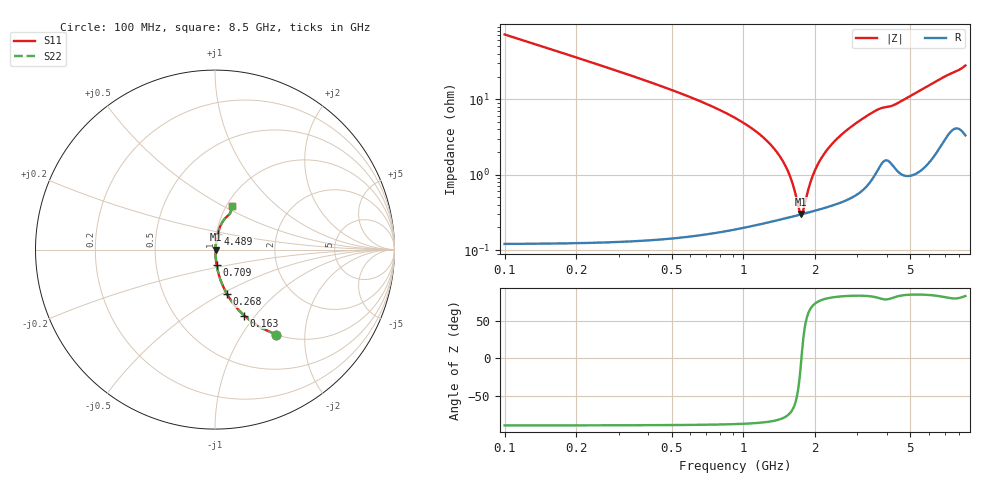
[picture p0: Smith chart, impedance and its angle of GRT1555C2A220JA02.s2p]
!Murata Part Number: GRT1555C2A220JA02
!These Parameters are Measured in Series Mode Connection
!Data Generated on Jun 19, 2026
!  o--ll--o
!Port1  Port2
!  o------o
!Operation Temp=25[degC], DC Bias Voltage=0[V]
!Freq. Start=100[MHz] Stop=9[GHz] 401[Steps]
# Hz S RI R 50
!Freq.(Hz) S11(Real) S11(Imag) S21(Real) S21(Imag) S12(Real) S12(Imag) S22(Real) S22(Imag)
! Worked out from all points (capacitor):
!   401 points, 100 MHz to 8.5 GHz, reference 50 ohm
!   read as one part in series: C = 22 pF near 142 MHz
!   lowest |Z| = 302 mohm at 1.738 GHz (marker M1)
!   series resonance near 1.749 GHz, so ESL is about 380 pH
!   S11 on the Smith chart (normalised r, x): 100 MHz: 1.00, -1.44; 163 MHz: 1.00, -0.88; 268 MHz: 1.00, -0.53; 709 MHz: 1.00, -0.17; 4.489 GHz: 1.02, +0.18; 8.5 GHz: 1.07, +0.56
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1e8  0.3423 -0.4736  0.6577 0.4736  0.6577 0.4736  0.3423 -0.4736
1.63e8  0.1628 -0.3678  0.8372 0.3678  0.8372 0.3678  0.1628 -0.3678
2.68e8  0.066 -0.2458  0.934 0.2458  0.934 0.2458  0.066 -0.2458
4.57e8  0.0226 -0.1439  0.9774 0.1439  0.9774 0.1439  0.0226 -0.1439
7.09e8  0.00879 -0.0843  0.9912 0.0843  0.9912 0.0843  0.00879 -0.0843
1.234e9  0.00314 -0.0293  0.9969 0.0293  0.9969 0.0293  0.00314 -0.0293
1.507e9  0.0028 -0.0123  0.9972 0.0123  0.9972 0.0123  0.0028 -0.0123
1.591e9  0.00282 -0.00783  0.9972 0.00783  0.9972 0.00783  0.00282 -0.00783
1.696e9  0.00291 -0.00255  0.9971 0.00255  0.9971 0.00255  0.00291 -0.00255
1.738e9  0.00296 -0.000534  0.997 0.000534  0.997 0.000534  0.00296 -0.000534
1.78e9  0.00302 0.00144  0.997 -0.00144  0.997 -0.00144  0.00302 0.00144
1.885e9  0.0032 0.00619  0.9968 -0.00619  0.9968 -0.00619  0.0032 0.00619
1.969e9  0.00338 0.00984  0.9966 -0.00984  0.9966 -0.00984  0.00338 0.00984
2.158e9  0.00388 0.0176  0.9961 -0.0176  0.9961 -0.0176  0.00388 0.0176
2.473e9  0.00498 0.0297  0.995 -0.0297  0.995 -0.0297  0.00498 0.0297
2.914e9  0.00725 0.0456  0.9928 -0.0456  0.9928 -0.0456  0.00725 0.0456
3.607e9  0.0155 0.0689  0.9845 -0.0689  0.9845 -0.0689  0.0155 0.0689
4.3e9  0.0188 0.0813  0.9812 -0.0813  0.9812 -0.0813  0.0188 0.0813
4.489e9  0.0183 0.0878  0.9817 -0.0878  0.9817 -0.0878  0.0183 0.0878
5.707e9  0.0305 0.1334  0.9695 -0.1334  0.9695 -0.1334  0.0305 0.1334
7.114e9  0.0676 0.1847  0.9324 -0.1847  0.9324 -0.1847  0.0676 0.1847
8.5e9  0.0973 0.2427  0.9027 -0.2427  0.9027 -0.2427  0.0973 0.2427
